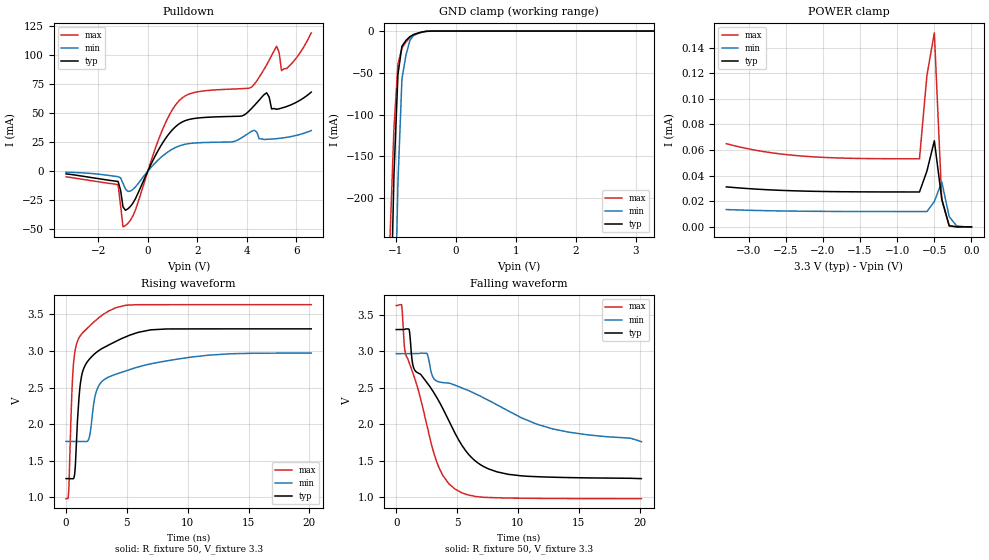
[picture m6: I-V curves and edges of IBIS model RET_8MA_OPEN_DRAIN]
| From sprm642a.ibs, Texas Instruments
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|   Model Cell RET_8MA_OPEN_DRAIN
|RET_8MA_OPEN_DRAIN
[Model]   RET_8MA_OPEN_DRAIN
Model_type   I/O_open_drain
Polarity   Inverting
Enable   Active-Low
Vinl =  0.8
Vinh =  2
Cref =  15.0000pF
Rref =  100.0000M
Vref =  0V
Vmeas =  1.65
C_comp   5.345208p   4.561426p   6.022817p
[Model Spec]
Vinl   0.8   0.8   0.8
Vinh   2   2   2
[Temperature Range]   25   155   -40
[Voltage Range]   3.3   2.97   3.63
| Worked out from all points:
|   slope of the pulldown table from 0 to 0.495 V, typ, clamps not added: 23.8 ohm
|   GND clamp passes 1 mA (typ) near -0.55 V on its own axis
|   rising waveform, R_fixture 50, V_fixture 3.3: 20-80 % time 1.11ns typ, 2.87ns min, 574ps max; typ from 1.26 V to 3.3 V
|   falling waveform, R_fixture 50, V_fixture 3.3: 20-80 % time 4.3ns typ, 8.66ns min, 2.62ns max; typ from 3.3 V to 1.26 V
| Nom Voltages:
|   BIASFET=3.3, VDD=1.2, VDDS=3.3, VSS=0
| Min Voltages:
|   BIASFET=2.97, VDD=1.08, VDDS=2.97, VSS=0
| Max Voltages:
|   BIASFET=3.63, VDD=1.32, VDDS=3.63, VSS=0
[POWER_clamp]
|   voltage   I(typ)   I(min)   I(max)
-3.3V     31.22uA    13.5uA     64.95uA
-2.8V     29.13uA    12.67uA    58.77uA
-2.3V     27.98uA    12.22uA    55.36uA
-1.7V     27.4uA     12.01uA    53.62uA
-700mV    27.24uA    11.95uA    53.12uA
-600mV    43.52uA    11.94uA    118.2uA
-500mV    67.2uA     19.79uA    151.5uA
-400mV    21.58uA    35.09uA    21.1uA
-300mV    927.4nA    7.958uA    611.4nA
-200mV    28.93nA    716.3nA    11.51nA
0V        696.9pA    39.48nA    568.3pA
[Pulldown]
|   voltage   I(typ)   I(min)   I(max)
-3.3V     -2.325mA   -885.1uA   -4.829mA
-1.2V     -8.9mA     -4.742mA   -11.78mA
-1V       -30.94mA   -10.56mA   -48.07mA
-900mV    -33.77mA   -15.53mA   -46.9mA
-500mV    -23.82mA   -13.61mA   -33.55mA
600mV     24.46mA    13.16mA    36.18mA
1.3V      41.39mA    22.04mA    61.62mA
4.2V      54.39mA    34.49mA    72.77mA
4.8V      67.66mA    27.49mA    91.8mA
5.2V      53.41mA    28.11mA    107.8mA
5.4V      54.46mA    28.58mA    86.79mA
6.6V      68.25mA    35.07mA    119.5mA
[GND_clamp]
|   voltage   I(typ)   I(min)   I(max)
-3.3V     -16.36A    -15.08A    -17.18A
-1.1V     -382.1mA   -717.8mA   -250.1mA
-1.033V   -173.3mA   -402.2mA   -116.4mA
-966.7mV  -52.02mA   -182.1mA   -39.81mA
-900mV    -18.21mA   -57.43mA   -20.34mA
-833.3mV  -11.36mA   -28.88mA   -13.17mA
-766.7mV  -6.618mA   -11.27mA   -8.134mA
-700mV    -3.983mA   -4.59mA    -5.247mA
-500mV    -328.3uA   -481.4uA   -374.5uA
-366.7mV  -15.94uA   -50.74uA   -14.83uA
3.3V      696.9pA    15.84uA    426.1pA
[Ramp]
| variable   typ   min   max
dV/dt_f  1.2310053/4.2984771n 0.72730904/8.6502749n  1.5950479/2.6227934n
dV/dt_r  1.2344632/3.7306612n 0.84436844/8.0035235n  1.5896397/2.2660664n
R_load = 50
[Rising Waveform]
R_fixture = 50
V_fixture = 3.3
V_fixture_min = 2.97
V_fixture_max = 3.63
|   time   V(typ)   V(min)   V(max)
0s        1.258V     1.765V     983.7mV
206.9ps   1.258V     1.765V     1.064V
516.9ps   1.255V     1.765V     2.584V
759.5ps   1.429V     1.765V     3.022V
1.01ns    2.244V     1.765V     3.161V
1.247ns   2.635V     1.765V     3.224V
1.901ns   2.884V     1.817V     3.334V
2.594ns   2.993V     2.493V     3.439V
6.952ns   3.286V     2.822V     3.63V
20.15ns   3.3V       2.97V      3.63V
[Falling Waveform]
R_fixture = 50
V_fixture = 3.3
V_fixture_min = 2.97
V_fixture_max = 3.63
|   time   V(typ)   V(min)   V(max)
0s        3.3V       2.97V      3.63V
446.6ps   3.3V       2.97V      3.635V
708.9ps   3.305V     2.97V      3.017V
1.059ns   3.303V     2.97V      2.846V
1.432ns   2.776V     2.97V      2.676V
2.538ns   2.573V     2.971V     1.97V
3.225ns   2.401V     2.606V     1.537V
4.853ns   1.874V     2.537V     1.112V
8.287ns   1.35V      2.268V     994.9mV
20.15ns   1.258V     1.765V     982.8mV
